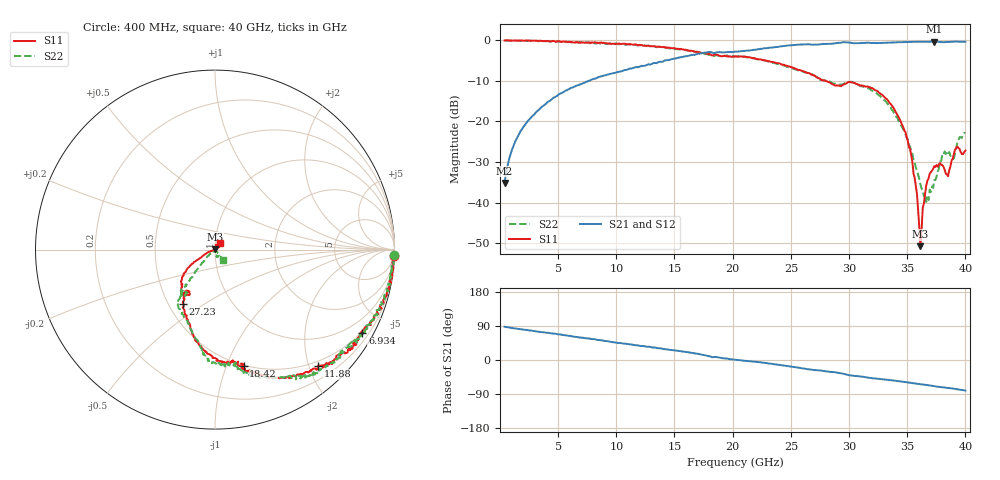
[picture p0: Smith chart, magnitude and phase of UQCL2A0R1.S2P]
! AVX Corporation
! Date:  10/27/06
! Part No:  UQCL2A0R1B
! Description:  Ultra Low ESR Microwave capacitors
! Mounting Orientation:  Horizontal
# GHZ S DB R 50
! Freq  |S11|  S11 Ph  |S21|  S21 Ph  |S12|  S12 Ph  |S22|  S22 Ph
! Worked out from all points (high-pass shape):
!   401 points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, 400 MHz to 40 GHz, reference 50 ohm
!   highest |S21| = -0.30 dB at 37.33 GHz (marker M1); lowest = -35.2 dB at 400 MHz (marker M2)
!   |S21| within 3 dB of the highest: 16.99 GHz to end of sweep
!   lowest |S11| = -50.8 dB at 36.14 GHz (marker M3), VSWR 1.01, Z = 49.9 + j0.263 ohm
!   |S11| at or under -10 dB: 28 GHz to end of sweep
!   |S22| runs from -39.9 to 0.0 dB; largest |S21 - S12| = 0.015
!   S11 on the Smith chart (normalised r, x): 400 MHz: 2, -56; 6.934 GHz: 0.44, -3.74; 11.88 GHz: 0.42, -2.15; 18.42 GHz: 0.49, -1.15; 27.23 GHz: 0.59, -0.41; 40 GHz: 1.05, +0.07
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0.4  -0.01 -2.0  -35.17 87.7  -35.21 87.4  -0.01 -1.8
1.192  -0.01 -6.6  -25.73 83.6  -25.81 83.4  -0.11 -5.0
2.38  -0.01 -10.5  -19.93 78.7  -20.01 78.3  -0.14 -11.5
6.934  -0.50 -29.6  -10.81 59.4  -10.86 59.4  -0.50 -29.4
7.033  -0.55 -29.9  -10.68 58.6  -10.66 59.7  -0.39 -29.5
11.884  -1.26 -48.5  -6.64 38.3  -6.54 37.9  -1.12 -53.3
13.666  -1.51 -57.6  -5.31 30.9  -5.31 30.3  -1.57 -59.2
18.418  -3.48 -76.2  -3.12 7.9  -3.17 8.0  -3.80 -79.5
20.2  -3.91 -82.3  -2.77 0.8  -2.81 0.7  -4.01 -88.2
26.833  -8.51 -117.6  -1.02 -25.8  -0.99 -25.7  -8.32 -121.8
27.229  -9.14 -120.6  -1.05 -27.0  -1.02 -27.2  -8.97 -125.4
30.496  -10.53 -129.2  -0.69 -42.1  -0.74 -42.3  -10.52 -129.8
33.466  -15.35 -146.2  -0.55 -52.9  -0.64 -52.8  -16.22 -132.0
35.05  -24.79 -155.5  -0.37 -59.2  -0.36 -59.5  -24.40 -138.3
35.545  -32.89 -163.0  -0.35 -61.4  -0.35 -61.2  -29.62 -140.8
36.139  -50.76 114.5  -0.36 -63.9  -0.37 -64.1  -35.47 -124.1
36.634  -35.80 32.8  -0.33 -65.8  -0.34 -65.8  -39.89 -88.0
37.327  -31.03 33.1  -0.30 -69.1  -0.30 -69.1  -34.44 -51.9
38.02  -30.75 36.4  -0.43 -72.0  -0.43 -72.3  -28.16 -55.4
38.515  -33.51 64.9  -0.39 -73.5  -0.40 -73.6  -27.82 -76.1
38.911  -29.22 81.6  -0.33 -75.2  -0.32 -75.3  -29.32 -72.8
40  -27.19 53.9  -0.33 -80.6  -0.34 -80.9  -22.82 -54.4
